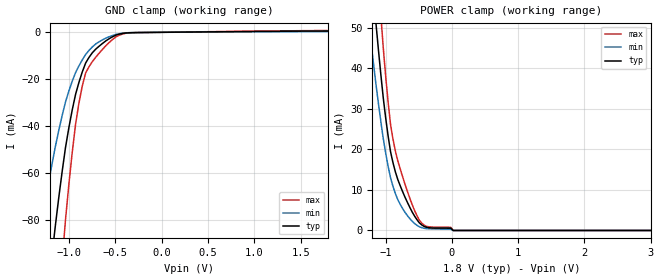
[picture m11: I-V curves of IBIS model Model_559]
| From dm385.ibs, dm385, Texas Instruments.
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| Model based on original model for BCSHTLTCSCDDVPBFZ_SSDHV
|   Sub model DIFF_LVCMOS_PD_ON_5PER_1P8
[model]   Model_559
|[Description]  [1.8V-INPUT-PD-X, IND, 5%]
|   Weak internal pull-down,Industrial temperature range (-40C to
|   125C, 25C nominal),5% power supply tolerance
|[Input Load]   PD
|[Output Drive]
|Voltage   1.8V
|Mode   INPUT
Model_type   Input
Polarity   Non-Inverting
Vinl =  0.63
Vinh =  1.17
C_comp   1.851324p   1.667199p   1.973575p
[Model Spec]
Vinl   0.63   0.5985   0.6615
Vinh   1.17   1.1115   1.2285
[Temperature Range]   25   125   -40
[Voltage Range]   1.8   1.71   1.89
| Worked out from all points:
|   GND clamp passes 1 mA (typ) near -0.47 V on its own axis
|   POWER clamp passes 1 mA (typ) near -0.42 V on its own axis
[POWER_clamp]
-1.8V     194.9mA    137mA      262.9mA
-1.255V   72.21mA    51.12mA    97.51mA
-1.218V   64.88mA    45.92mA    88.08mA
-1.145V   50.84mA    35.88mA    69.81mA
-1.073V   38.39mA    26.83mA    52.95mA
-1.036V   32.65mA    22.64mA    44.98mA
-927.3mV  19.46mA    13.02mA    26.21mA
-854.5mV  14.5mA     9.137mA    19.63mA
-672.7mV  6.948mA    3.681mA    9.678mA
-490.9mV  1.858mA    895.5uA    2.506mA
18.18mV   0A         0A         0A
3.6V      0A         0A         0A
[GND_clamp]
-1.8V     -346.1mA   -209.3mA   -568.3mA
-1.327V   -149.8mA   -89.05mA   -251mA
-1.291V   -135.7mA   -80.49mA   -227.6mA
-1.145V   -82.42mA   -48.7mA    -137.8mA
-1.073V   -59.53mA   -35.59mA   -98.08mA
-1.036V   -49.2mA    -29.76mA   -80.02mA
-927.3mV  -26.44mA   -17.17mA   -39.17mA
-854.5mV  -16.84mA   -11.72mA   -22.8mA
-818.2mV  -13.04mA   -9.437mA   -17.24mA
-672.7mV  -5.895mA   -4.018mA   -8.877mA
-381.8mV  -267.3uA   -214.4uA   -368.9uA
1.8V      561.9uA    351.4uA    768.3uA
